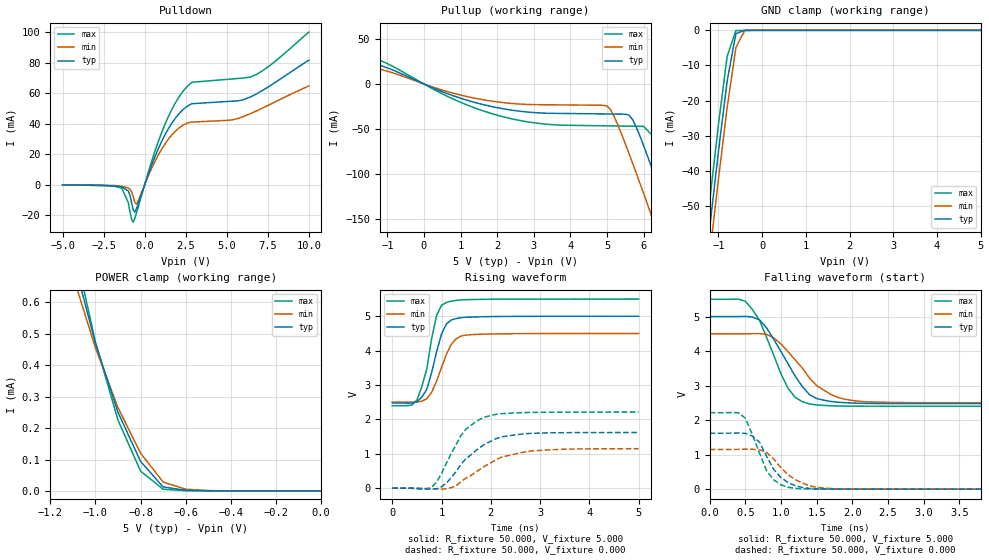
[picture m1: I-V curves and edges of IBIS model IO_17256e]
| IBIS file xc17256e.ibs created by s2ibis2 version 1.1
| North Carolina State University Electronics Research Laboratory  1995
[IBIS ver]   2.1
[File name]   xc17256e.ibs
[File Rev]   2.0
[Date]   Feb. 05, 1999
[Source]   Spice netlist
[Copyright]   Xilinx Inc. All right reserved
|   Component XC17256e_pd8
[Component]   XC17256e_pd8
[Manufacturer]   Xilinx Inc.
[Package]
| variable   typ   min   max
R_pkg   56.00m   52.000m   60.00m
L_pkg   2.265nH   2.100nH   2.430nH
C_pkg   0.275pF   0.260pF   0.290pF
[Pin]  signal_name   model_name   R_pin   L_pin   C_pin
| in   dataout   input   NA   NA   NA
| oe   enowb   enable   NA   NA   NA
vdd   vdd   POWER   NA   NA   NA
vgnd   gnd   GND   NA   NA   NA
io   data   IO_17256e   NA   NA   NA
| Models and submodels in the file (1): IO_17256e (I/O)
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|   Model IO_17256e
[Model]   IO_17256e
Model_type   I/O
Polarity   Non-Inverting
Enable   Active-High
Vinl =   0.800V
Vinh =   2.000V
Vmeas =   2.500V
Cref =  50.000pF
Rref =   1.000M
Vref =  0.000V
C_comp   2.500pF   2.000pF   3.000pF
[Temperature Range]   50.000   100.000   0.000
[Voltage Range]   5.000V   4.500V   5.500V
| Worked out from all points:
|   slope of the pulldown table from 0 to 0.75 V, typ, clamps not added: 34.8 ohm
|   slope of the pullup table from 0 to 0.75 V, typ, clamps not added: 61 ohm
|   GND clamp passes 1 mA (typ) near -0.60 V on its own axis
|   POWER clamp passes 1 mA (typ) near -1.18 V on its own axis
|   rising waveform, R_fixture 50.000, V_fixture 5.000: 20-80 % time 281ps typ, 336ps min, 266ps max; typ from 2.48 V to 5 V
|   rising waveform, R_fixture 50.000, V_fixture 0.000: 20-80 % time 697ps typ, 832ps min, 543ps max; typ from 0 V to 1.62 V
|   falling waveform, R_fixture 50.000, V_fixture 5.000: 20-80 % time 445ps typ, 528ps min, 375ps max; typ from 5 V to 2.48 V
|   falling waveform, R_fixture 50.000, V_fixture 0.000: 20-80 % time 292ps typ, 375ps min, 273ps max; typ from 1.62 V to 0 V
[Pulldown]
| voltage   I(typ)   I(min)   I(max)
-5V       -200uA     -200uA     -200uA
-1.4V     -1.52mA    -1.05mA    -2.31mA
-1V       -4.24mA    -2.23mA    -11.68mA
-700mV    -16.52mA   -7.72mA    -24.62mA
-500mV    -15.7mA    -12.73mA   -18.48mA
1.1V      29.76mA    24.43mA    35.92mA
1.8V      42.57mA    34.29mA    52.27mA
2.5V      50.63mA    39.89mA    63.28mA
2.9V      53.06mA    41.02mA    67.13mA
5.3V      54.69mA    42.43mA    69.25mA
6.8V      59.43mA    48.29mA    72.2mA
10V       81.64mA    64.73mA    100mA
[Pullup]
| voltage   I(typ)   I(min)   I(max)
-5V       43.92mA    29.41mA    61.71mA
-3.4V     41.05mA    30.39mA    53.53mA
-1.8V     28.3mA     22.28mA    35.96mA
2.1V      -26.98mA   -20.33mA   -35.61mA
5V        -33.2mA    -24.42mA   -46.35mA
5.2V      -33.3mA    -36.34mA   -46.47mA
5.7V      -39.46mA   -87.77mA   -46.75mA
6V        -68.19mA   -121mA     -46.93mA
6.4V      -112mA     -167mA     -63.73mA
6.8V      -158mA     -213mA     -107mA
7.2V      -205mA     -260mA     -153mA
10V       -542mA     -591mA     -495mA
[GND_clamp]
| voltage   I(typ)   I(min)   I(max)
-5V       -506mA     -507mA     -507mA
-1.4V     -78.45mA   -85.98mA   -71.13mA
-1.2V     -56.14mA   -63.89mA   -48.55mA
-1V       -34.52mA   -42.36mA   -26.81mA
-800mV    -14.4mA    -21.94mA   -7.379mA
-600mV    -951uA     -4.891mA   -78.38uA
-400mV    -3.259uA   -75.77uA   -196nA
5V        535pA      1.161uA    58.62pA
[POWER_clamp]
| voltage   I(typ)   I(min)   I(max)
-5V       23.72mA    17.68mA    31.13mA
-1.1V     744uA      686uA      797uA
-1V       470uA      455uA      474uA
-900mV    250uA      265uA      225uA
-800mV    93.83uA    120uA      63.03uA
-700mV    12.61uA    28.28uA    5.367uA
-600mV    2.134uA    5.354uA    605nA
-500mV    334nA      1.161uA    62.96nA
0V        535pA      6.967nA    70.34pA
[Ramp]
| variable   typ   min   max
dV/dt_r   0.972/0.696n   0.689/0.839n   1.328/0.555n
dV/dt_f   1.514/0.443n   1.198/0.530n   1.861/0.369n
R_load = 50.000
[Rising Waveform]
R_fixture = 50.000
V_fixture = 5.000
V_fixture_min = 4.500
V_fixture_max = 5.500
L_fixture = 0.000H
C_fixture = 0.000F
| time   V(typ)   V(min)   V(max)
0s        2.477V     2.504V     2.399V
400ps     2.477V     2.5V       2.421V
500ps     2.514V     2.503V     2.567V
700ps     2.875V     2.6V       3.47V
900ps     3.974V     3.117V     5.029V
1ns       4.487V     3.513V     5.316V
1.1ns     4.778V     3.897V     5.404V
1.3ns     4.935V     4.351V     5.461V
1.5ns     4.971V     4.454V     5.482V
5ns       5V         4.5V       5.5V
[Rising Waveform]
R_fixture = 50.000
V_fixture = 0.000
V_fixture_min = 0.000
V_fixture_max = 0.000
L_fixture = 0.000H
C_fixture = 0.000F
| time   V(typ)   V(min)   V(max)
0s        0V         0V         0V
800ps     -27.88mV   -14.58mV   31.24mV
900ps     -13.23mV   -21.48mV   177mV
1.1ns     151mV      -15.45mV   736mV
1.4ns     707mV      194mV      1.548V
1.7ns     1.1V       474mV      1.939V
1.9ns     1.295V     658mV      2.076V
2.2ns     1.488V     895mV      2.166V
2.8ns     1.594V     1.079V     2.204V
5ns       1.62V      1.149V     2.214V
[Falling Waveform]
R_fixture = 50.000
V_fixture = 5.000
V_fixture_min = 4.500
V_fixture_max = 5.500
L_fixture = 0.000H
C_fixture = 0.000F
| time   V(typ)   V(min)   V(max)
0s        5V         4.5V       5.5V
500ps     5.005V     4.5V       5.442V
700ps     4.902V     4.506V     4.886V
900ps     4.337V     4.381V     3.868V
1.1ns     3.628V     3.98V      2.918V
1.2ns     3.269V     3.742V     2.659V
1.4ns     2.736V     3.217V     2.467V
1.7ns     2.54V      2.742V     2.416V
2.1ns     2.488V     2.545V     2.403V
5ns       2.477V     2.504V     2.399V
[Falling Waveform]
R_fixture = 50.000
V_fixture = 0.000
V_fixture_min = 0.000
V_fixture_max = 0.000
L_fixture = 0.000H
C_fixture = 0.000F
| time   V(typ)   V(min)   V(max)
0s        1.62V      1.15V      2.215V
400ps     1.626V     1.153V     2.214V
500ps     1.618V     1.157V     2.058V
700ps     1.359V     1.138V     1.037V
800ps     944mV      1.06V      524mV
900ps     566mV      866mV      269mV
1.1ns     191mV      417mV      54.56mV
1.4ns     21.27mV    95.59mV    5.971mV
1.7ns     4.128mV    19.27mV    1.848mV
5ns       -14.78uV   40.05uV    21.38uV
